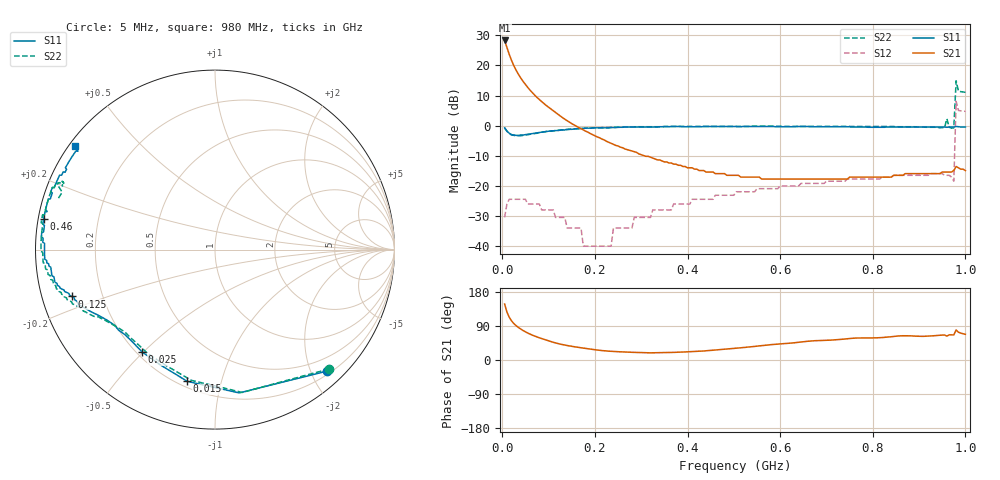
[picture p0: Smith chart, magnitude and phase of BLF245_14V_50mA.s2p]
! Filename:  BLF245_14V_50mA.s2p
! Philips part #: BLF245  !date: 22-05-2003
!Vdd=14V ; Idq=50 mA
!D:\Vee measurements\measurement data\VDMOST\BLF245\14V_50mA_#1
# HZ S MA R 50
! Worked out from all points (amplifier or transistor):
!   200 points, 5 MHz to 1 GHz, reference 50 ohm
!   highest |S21| = 28.3 dB at 5 MHz (marker M1)
!   |S21| within 3 dB of that: start of sweep to 11.41 MHz
!   unconditionally stable (mu >= 1): 174.1 MHz to 199.1 MHz; 200.6 MHz to 236.2 MHz; 602.5 MHz to 955.6 MHz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
!   at 170 MHz: K = 0.22, MSG = 16.5 dB, |S12| = -34.0 dB
!   at 505 MHz: K = 0.82, MSG = 2.7 dB, |S12| = -21.9 dB
!   at 1 GHz: K = -2.26, MSG = -9.8 dB, |S12| = 4.8 dB
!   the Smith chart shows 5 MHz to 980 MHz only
!   S11 on the Smith chart (normalised r, x): 5 MHz: 0.26, -2.25; 15 MHz: 0.23, -0.78; 25 MHz: 0.22, -0.50; 125 MHz: 0.09, -0.16; 460 MHz: 0.02, +0.09; 980 MHz: 0.02, +0.33
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5000000  0.92 -47.4  25.96 147.8  0.03 58.6  0.92 -46.3
1e7  0.81 -80.4  19.77 126.7  0.05 37.7  0.81 -79.2
1.5e7  0.75 -101.9  15.25 112.9  0.06 24.4  0.74 -100.3
2e7  0.71 -116.0  12.1 103.2  0.06 15.8  0.7 -113.5
2.5e7  0.7 -125.4  9.87 96.0  0.06 9.2  0.69 -122.9
4e7  0.7 -140.1  6.16 81.5  0.06 -3.7  0.68 -137.5
6e7  0.73 -148.6  3.88 68.2  0.05 -14.1  0.72 -146.0
8.5e7  0.78 -154.2  2.51 56.6  0.04 -22.0  0.78 -152.1
1.25e8  0.84 -161.9  1.45 41.9  0.03 -27.5  0.85 -159.2
1.75e8  0.9 -167.9  0.85 31.4  0.01 -8.8  0.9 -165.6
3.4e8  0.96 177.6  0.27 19.3  0.04 85.7  0.96 -178.8
4.6e8  0.97 170.0  0.16 26.4  0.07 86.4  0.97 174.8
5.05e8  0.97 167.5  0.15 31.1  0.08 84.6  0.97 172.7
6.7e8  0.96 158.6  0.13 50.5  0.11 81.5  0.97 165.8
8.35e8  0.95 151.1  0.14 60.8  0.14 80.3  0.97 159.4
9.5e8  0.95 144.9  0.17 65.8  0.16 74.2  0.93 155.9
9.6e8  0.94 144.3  0.17 63.0  0.15 -142.4  1.3 -171.4
9.65e8  0.95 144.2  0.17 66.4  0.15 75.0  0.94 158.0
9.75e8  0.95 143.7  0.18 66.2  0.12 69.6  0.92 162.5
9.8e8  0.97 143.3  0.21 79.3  2.54 41.9  5.56 44.3
9.85e8  0.96 143.2  0.2 73.3  1.79 42.9  3.73 48.8
1e9  0.95 142.7  0.18 67.8  1.73 41.9  3.58 47.5
